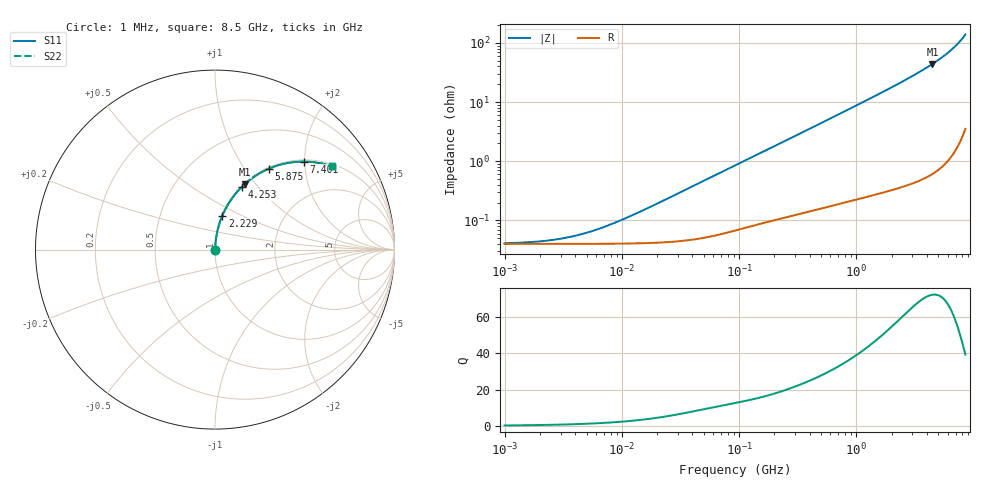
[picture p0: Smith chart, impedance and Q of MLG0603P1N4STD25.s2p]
! S-Parameter Data Generated by TDK Corporation
! Copyright(C) 2025 TDK Corporation.
! All Rights Reserved.
! TDK P/N: MLG0603P1N4STD25 (SMD / SMT Inductor (Coil))
! Property: L=1.4nH at 500MHz
! Size(LxWxT): 0.6x0.3x0.3mm
! Model Type: s2p (Touchstone File Format Version 1.0)
! Frequency: DC=Yes Start=1MHz Stop=8500MHz 198points Log-sweep
! Model Generated on Feb. 6, 2025
! Terms and conditions regarding TDK Simulation Models:
! 1)This simulation model is being provided solely for informational
!  purposes. Please refer to the specifications of the products in
!  terms of detailed characteristics of such products.
! 2)In no event shall TDK Corporation of any of its subsidiaries be
!  liable for any loss or damage arising, directly or indirectly,
!  from any information contained in this simulation model, including,
!  but not limited to loss or damages arising from any inaccuracies,
!  omissions or errors in connection with such information.
! 3)Any and all copyrights on this simulation model are owned by
!  TDK Corporation.  Duplication or redistribution of this simulation
!  model without prior written permission from TDK Corporation
!  is prohibited.
! 4)This simulation model is subject to any modification or change
!  without any prior notice.
! 5)Neither TDK Corporation nor any of its subsidiaries shall make any
!  warranty, express or implied, including but not limited to the
!  correctness, implied warranties of merchantability and fitness for
!  a particular purpose with respect to this simulation models.
! 6)The use of this simulation model shall be deemed to have consented
!  to the terms and conditions hereof.
! Port Assignments:
!  1 ---@@@--- 2
! Applicable Conditions:
!  Temperature = 25 degC
!  DC Bias Current = 0 A
!  Small Signal Operation
# Hz S MA R 50
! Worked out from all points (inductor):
!   197 points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, 1 MHz to 8.5 GHz, reference 50 ohm
!   read as one part in series: L = 1.49 nH near 13.26 MHz
!   highest Q = 72.3 at 4.454 GHz (marker M1), where L = 1.57 nH
!   S11 on the Smith chart (normalised r, x): 1 MHz: 1.00, +0.00; 2.229 GHz: 1.01, +0.40; 4.253 GHz: 1.01, +0.83; 5.875 GHz: 1.02, +1.30; 7.401 GHz: 1.04, +1.98; 8.5 GHz: 1.07, +2.77
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1000000  0.0004107 13.2  0.9996 -0.0  0.9996 -0.0  0.0004107 13.2
1661608  0.0004293 21.3  0.9996 -0.0  0.9996 -0.0  0.0004293 21.3
2403882  0.0004593 29.4  0.9996 -0.0  0.9996 -0.0  0.0004593 29.4
3320851  0.0005073 37.9  0.9996 -0.0  0.9996 -0.0  0.0005073 37.9
4587603  0.0005881 47.0  0.9996 -0.0  0.9996 -0.0  0.0005881 47.0
6337562  0.0007174 55.9  0.9996 -0.0  0.9996 -0.0  0.0007174 55.9
8755050  0.0009147 63.8  0.9996 -0.0  0.9996 -0.0  0.0009147 63.8
1.26661e7  0.001255 71.0  0.9996 -0.1  0.9996 -0.1  0.001255 71.0
2.10461e7  0.002015 77.8  0.9996 -0.1  0.9996 -0.1  0.002015 77.8
9.219544e7  0.008475 85.0  0.9993 -0.5  0.9993 -0.5  0.008475 85.0
4.229561e8  0.03725 85.6  0.9979 -2.1  0.9979 -2.1  0.03725 85.6
9.708683e8  0.08448 83.7  0.9942 -4.8  0.9942 -4.8  0.08448 83.7
1.940355e9  0.1687 79.2  0.9825 -9.7  0.9825 -9.7  0.1687 79.2
2.228565e9  0.1942 77.8  0.9776 -11.2  0.9776 -11.2  0.1942 77.8
3.224109e9  0.284 72.6  0.9546 -16.5  0.9546 -16.5  0.284 72.6
4.253027e9  0.3809 66.8  0.9193 -22.4  0.9193 -22.4  0.3809 66.8
4.453958e9  0.4003 65.6  0.9108 -23.6  0.9108 -23.6  0.4003 65.6
5.115526e9  0.4655 61.5  0.8786 -27.7  0.8786 -27.7  0.4655 61.5
5.87536e9  0.5421 56.3  0.8324 -32.8  0.8324 -32.8  0.5421 56.3
6.748056e9  0.6312 49.9  0.7653 -39.1  0.7653 -39.1  0.6312 49.9
7.400733e9  0.697 44.7  0.7041 -44.2  0.7041 -44.2  0.697 44.7
8.5e9  0.8011 35.3  0.5786 -53.2  0.5786 -53.2  0.8011 35.3
